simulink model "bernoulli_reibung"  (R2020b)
settings: Solver=VariableStepAuto  StartTime=0.0  StopTime=40  RelTol=1e-3
model workspace (MAT data in the model file):
  D = 0.5
  H = 12
  L = 600
  g = 9.81
  lambda = 0.03
  zeta_ein = 0.5

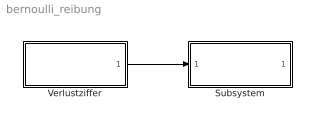
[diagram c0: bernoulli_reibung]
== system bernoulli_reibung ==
  Subsystem : Subsystem
  Verlustziffer : Subsystem
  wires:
  Verlustziffer/1(Out1) -> Subsystem/1(In1)

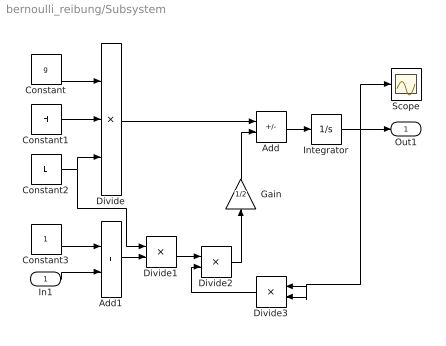
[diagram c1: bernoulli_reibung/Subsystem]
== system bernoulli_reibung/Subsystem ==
  In1 : Inport
  Add : Sum  Inputs=+-
  Add1 : Sum
  Constant : Constant  Value=g
  Constant1 : Constant  Value=H
  Constant2 : Constant  Value=L
  Constant3 : Constant
  Divide : Product  Inputs=**/
  Divide1 : Product  Inputs=/*
  Divide2 : Product  Inputs=**
  Divide3 : Product  Inputs=**
  Gain : Gain  Gain=1/2
  Integrator : Integrator
  Scope : Scope
  Out1 : Outport
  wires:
  Constant/1 -> Divide/1
  Constant1/1 -> Divide/2
  Constant2/1 -> Divide1/1, Divide/3
  Constant3/1 -> Add1/1
  In1/1 -> Add1/2
  Add1/1 -> Divide1/2
  Divide1/1 -> Divide2/1
  Divide/1 -> Add/1
  Divide2/1 -> Gain/1
  Add/1 -> Integrator/1
  Integrator/1 -> Scope/1, Out1/1, Divide3/2, Divide3/1
  Gain/1 -> Add/2
  Divide3/1 -> Divide2/2

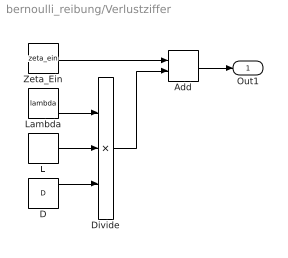
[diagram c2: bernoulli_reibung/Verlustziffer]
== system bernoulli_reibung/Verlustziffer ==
  Add : Sum
  D : Constant  Value=D
  Divide : Product  Inputs=**/
  L : Constant  Value=L
  Lambda : Constant  Value=lambda
  Zeta_Ein : Constant  Value=zeta_ein
  Out1 : Outport
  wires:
  Lambda/1 -> Divide/1
  L/1 -> Divide/2
  D/1 -> Divide/3
  Zeta_Ein/1 -> Add/1
  Divide/1 -> Add/2
  Add/1 -> Out1/1
